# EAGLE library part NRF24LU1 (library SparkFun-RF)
Nordic nRF24LU1+ Single-Chip 2.4GHz Transceiver w/ USB Microcontroller and Flash Nordic’s nRF24LU1+ is a complete system-on-chip wireless transceiver. The nRF24LU1+ features a fully integrated USB 2.0 compliant device controller, which makes this chip a great choice for a compact wireless USB dongle. The nRF24LU1+ is compatible with our nRF24L01+ 2.4GHz RF transceivers as well. Additional features include an 8-bit application microcontroller, 32 kB flash memory, 6 GPIO pins, SPI and UART support, and up to 2Mbps on air data rates. SparkFun Products 2.4GHz Transceiver IC - nRF24LU1+ (COM-09525)
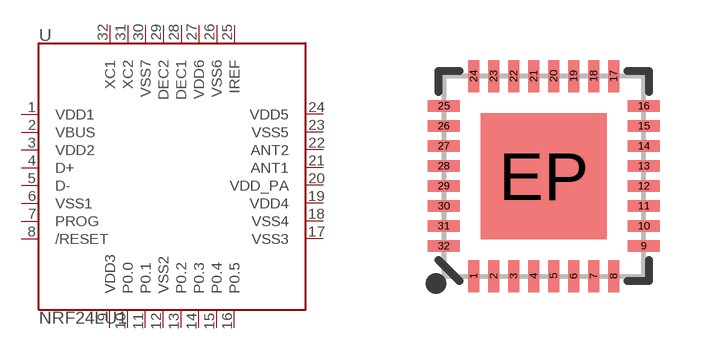
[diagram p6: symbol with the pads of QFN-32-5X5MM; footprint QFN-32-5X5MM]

Designator prefix -

## NRF24LU1 (PROD_ID: IC-09045)  [QFN-32-5X5MM]
1  VDD1
2  VBUS
3  VDD2
4  D+
5  D-
6  VSS1
7  PROG
8  /RESET
9  VDD3
10  P0.0
11  P0.1
12  VSS2
13  P0.2
14  P0.3
15  P0.4
16  P0.5
17  VSS3
18  VSS4
19  VDD4
20  VDD_PA
21  ANT1
22  ANT2
23  VSS5
24  VDD5
25  IREF
26  VSS6
27  VDD6
28  DEC1
29  DEC2
30  VSS7
31  XC2
32  XC1

## Footprint QFN-32-5X5MM (pad centres in mm)
QFN 32-Pin w/ Thermal Pad - 5.0 x 5.0 mm Used by nRF24LU1 and nRF24LE1 Datasheet Example
smd 0.285 x 0.8: 1 -1.75,-2.5; 2 -1.25,-2.5; 3 -0.75,-2.5; 4 -0.25,-2.5; 5 0.25,-2.5; 6 0.75,-2.5; 7 1.25,-2.5; 8 1.75,-2.5; 17 1.75,2.5; 18 1.25,2.5; 19 0.75,2.5; 20 0.25,2.5; 21 -0.25,2.5; 22 -0.75,2.5; 23 -1.25,2.5; 24 -1.75,2.5
smd 0.8 x 0.285: 9 2.5,-1.75; 10 2.5,-1.25; 11 2.5,-0.75; 12 2.5,-0.25; 13 2.5,0.25; 14 2.5,0.75; 15 2.5,1.25; 16 2.5,1.75; 25 -2.5,1.75; 26 -2.5,1.25; 27 -2.5,0.75; 28 -2.5,0.25; 29 -2.5,-0.25; 30 -2.5,-0.75; 31 -2.5,-1.25; 32 -2.5,-1.75
smd 3.15 x 3.15: EP 0,0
